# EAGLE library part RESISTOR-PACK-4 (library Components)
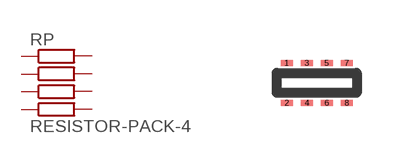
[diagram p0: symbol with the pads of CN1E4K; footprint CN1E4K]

Designator prefix RP

## RESISTOR-PACK-4  [CN1E4K]
1  1  pas
2  2  pas
3  3  pas
4  4  pas
5  5  pas
6  6  pas
7  7  pas
8  8  pas

## Footprint CN1E4K (pad centres in mm)
4 Resistor Pack
smd 0.3 x 0.15: 1 0,0.5; 2 0,-0.5; 3 0.5,0.5; 4 0.5,-0.5; 5 1,0.5; 6 1,-0.5; 7 1.5,0.5; 8 1.5,-0.5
